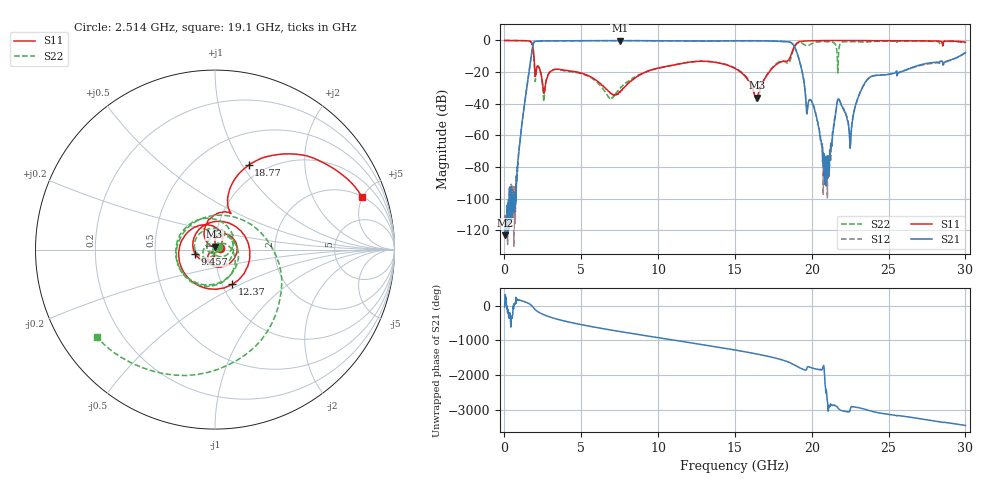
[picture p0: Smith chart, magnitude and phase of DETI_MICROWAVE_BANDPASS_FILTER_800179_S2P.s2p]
! 12/17/2019 3:59:58 PM
! \\DETI-AD\SERVEUR COMMUN\8 - PRODUITS FINIS\00\179 - BPF-SS-1200-20-2000-18000-21000-20-SF-SF\81 - PV\000 001.S2P
! CHANNEL.1
! TR.MEASUREMENT
! CORRECTED.DATA
# GHZ S RI R 50.0
! FREQ.GHZ  S11RE  S11IM  S21RE  S21IM  S12RE  S12IM  S22RE  S22IM
!; PortSelection: Port_12
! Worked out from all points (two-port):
!   2001 points, 10 MHz to 30 GHz, reference 50 ohm
!   highest |S21| = -0.10 dB at 7.508 GHz (marker M1); lowest = -123.0 dB at 25 MHz (marker M2)
!   |S21| within 3 dB of the highest: 1.853 GHz to 18.83 GHz (16.97 GHz wide, 164 % of centre)
!   lowest |S11| = -36.1 dB at 16.41 GHz (marker M3), VSWR 1.03, Z = 49.7 + j1.55 ohm
!   |S11| at or under -10 dB: 1.918 GHz to 18.62 GHz (16.7 GHz wide, 163 % of centre)
!   |S22| runs from -38.7 to 0.0 dB; largest |S21 - S12| = 0.014
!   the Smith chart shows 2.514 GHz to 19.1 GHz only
!   S11 on the Smith chart (normalised r, x): 2.514 GHz: 1.06, +0.02; 9.457 GHz: 0.80, -0.04; 12.37 GHz: 1.12, -0.45; 18.77 GHz: 0.84, +1.07; 19.1 GHz: 2.05, +4.94
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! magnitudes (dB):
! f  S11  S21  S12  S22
! 10 MHz  0.0  -122.8  -112.6  0.0
! 25 MHz  0.0  -123.0  -115.4  0.0
! 789.7 MHz  0.0  -89.3  -89.1  0.0
! 1.824 GHz  -2.9  -4.5  -4.5  -3.1
! 2.514 GHz  -30.0  -0.3  -0.3  -32.7
! 5.018 GHz  -20.7  -0.2  -0.2  -21.0
! 7.508 GHz  -32.6  -0.1  -0.1  -30.5
! 9.457 GHz  -18.9  -0.1  -0.1  -19.1
! 10.01 GHz  -17.4  -0.2  -0.2  -17.6
! 12.37 GHz  -13.3  -0.3  -0.3  -13.3
! 15.01 GHz  -17.6  -0.2  -0.2  -17.4
! 16.41 GHz  -36.1  -0.2  -0.2  -38.2
! 18.77 GHz  -5.9  -2.4  -2.4  -6.9
! 19.1 GHz  -1.2  -9.5  -9.5  -1.7
! 19.67 GHz  -0.3  -45.4  -45.5  -3.4
! 20.01 GHz  -0.2  -39.0  -38.6  -1.9
! 21 GHz  0.0  -75.9  -75.5  -0.7
! 21.74 GHz  0.0  -36.8  -36.7  -9.5
! 22.52 GHz  0.0  -66.6  -65.5  -0.7
! 23.51 GHz  -0.1  -26.1  -26.2  -0.9
! 25.01 GHz  -0.1  -21.4  -21.3  -0.4
! 30 GHz  -1.1  -7.7  -7.7  -1.4
